| IBIS file 3599z.ibs created by s2ibis2 version 1.1
| North Carolina State University Electronics Research Laboratory  1995
[IBIS ver]   2.1
[File name]   v3599bc.ibs
[File Rev]   2.0
|1.0 : Original Version - Wei-Ling Chang
|2.0 : Replaced I/O and Input models with 70V659 ADC models - S.Kashyap 06/30/04
[Source]   Integrated Device Technology, Inc.
[Notes]   1.Temperatures: typ=25C, min=100C, max=0C 2.RRmp rates based
   on 50 ohm load. 3. Both inpad and iopad have 2 models each.
   (JTAG pins have one model.)
   iopad: standard 3.3V I/O model
   inpad: standard 3.3V input pad model
   iopad25: For 2.5V I/O supply
   inpad25: For 2.5V I/O supply.
   To use 2.%V models at any port, use iopad25 and inpad25
   as the model definition in pin defie section of the IBIS
   file.  JTAG pins only have models for 3.3V I/O voltage.
[Disclaimer] Integrated Device Technology, Inc. ("IDT") hereby grants the
   user of this IBIS model a non-exclusive, nontransferable
   license to use this IBIS model under the following terms. The
   user is granted this license only to use the IBIS model and is
   not granted rights to sell, copy (except as needed to run the
   IBIS model), rent, lease or sub-license the IBIS model in
   whole or in part, or in modified form to anyone. The User may
   modify the IBIS model to suit its specific applications, but
   rights to derivative works and such modifications shall belong
   to IDT. This IBIS model is provided on an AS IS" basis and IDT
   makes absolutely no warranty with respect to the information
   contained herein. IDT DISCLAIMS AND CUSTOMER WAIVES ALL
   WARRANTIES, EXPRESS AND IMPLIED, INCLUDING WARRANTIES OF
   MERCHANTABILITY AND FITNESS FOR A PARTICULAR PURPOSE. THE
   ENTIRE RISK AS TO QUALITY AND PERFORMANCE IS WITH THE USER
   ACCORDINGLY, IN NO EVENT SHALL IDT BE LIABLE FOR ANY DIRECT OR
   INDIRECT DAMAGES, WHETHER IN CONTRACT OR TORT, INCLUDING ANY
   LOST PROFITS OR OTHER INCIDENTAL, CONSEQUENTIAL, EXEMPLARY, OR
   PUNITIVE DAMAGES ARISING OUT OF THE USE OR APPLICATION OF THE
   IBIS model. Further, IDT reserves the right to make changes
   without notice to any product herein to improve reliability,
   function, or design. IDT does not convey any license under
   patent rights or any other intellectual property rights,
   including those of third parties. IDT is not obligated to
   provide maintenance or support for the licensed IBIS model.
[Copyright]   Copyright 2004, Integrated Device Technology, Inc. all rights
   reserved
|   Component idt70v3599z
[Component]   idt70v3599z
[Manufacturer]   Integrated Device Technology
[Package]
| BGA (BC256)
| variable   typ   min   max
R_pkg   54.00m   48.00m   60.00m
L_pkg   2.48nH   2.20nH   2.75nH
C_pkg   0.46pF   0.41pF   0.51pF
[Pin]  signal_name   model_name   R_pin   L_pin   C_pin
C2   io19l   iopad
D2   io19r   iopad
D3   io20l   iopad
D1   io20r   iopad
D5   vddql   POWER
E7   vss   GND
E2   io21l   iopad
E1   io21r   iopad
E3   io22l   iopad
F2   io22r   iopad
D7   vddqr   POWER
E8   vss   GND
F1   io23l   iopad
F3   io23r   iopad
G2   io24l   iopad
G1   io24r   iopad
D6   vddql   POWER
F6   vss   GND
G3   io25l   iopad
H2   io25r   iopad
H1   io26l   iopad
H3   io26r   iopad
G4   vddqr   POWER
G5   vss   GND
D4   vdd   POWER
E5   vdd   POWER
G6   vss   GND
E4   vddql   POWER
C3   vss   GND
J3   io27r   iopad
J1   io27l   iopad
J2   io28r   iopad
K3   io28l   iopad
H4   vddqr   POWER
H5   vss   GND
K1   io29r   iopad
K2   io29l   iopad
L3   io30r   iopad
L1   io30l   iopad
J4   vddql   POWER
J5   vss   GND
L2   io31r   iopad
M3   io31l   iopad
M1   io32r   iopad
M2   io32l   iopad
L4   vddqr   POWER
L6   vss   GND
N3   io33r   iopad
N1   io33l   iopad
N2   io34r   iopad
P2   io34l   iopad
P1   io35r   iopad
R1   io35l   iopad
N4   vdd   POWER
M7   vss   GND
P4   a16r   inpad
R5   a15r   inpad
T5   a14r   inpad
P5   a13r   inpad
R6   a12r   inpad
T6   a11r   inpad
P6   a10r   inpad
R7   a9r   inpad
T7   a8r   inpad
P7   a7r   inpad
R8   be3r#   inpad
T8   be2r#   inpad
P8   be1r#   inpad
P9   be0r#   inpad
T9   ce1r   inpad
R9   ce0r#   inpad
N13   vdd   POWER
M12   vdd   POWER
M9   vss   GND
M10   vss   GND
P10   clkr   inpad
T10   oer#   inpad
R10   rwr#   inpad
P11   adsr#   inpad
T11   cntenr#   inpad
R11   repeatr#  inpad
P12   a6r   inpad
T12   a5r   inpad
R12   a4r   inpad
P13   a3r   inpad
T13   a2r   inpad
R13   a1r   inpad
T14   a0r   inpad
M11   vdd   POWER
M8   vss   GND
M6   vdd   POWER
P14   io0l   iopad
P15   io0r   iopad
N12   vddql   POWER
L11   vss   GND
P16   io1l   iopad
N15   io1r   iopad
N14   io2l   iopad
N16   io2r   iopad
N10   vddqr   POWER
L10   vss   GND
M15   io3l   iopad
M14   io3r   iopad
M16   io4l   iopad
L15   io4r   iopad
N11   vddql   POWER
L9   vss   GND
L14   io5l   iopad
L16   io5r   iopad
K15   io6l   iopad
K14   io6r   iopad
K13   vddqr   POWER
K12   vss   GND
K16   io7l   iopad
J15   io7r   iopad
J16   io8l   iopad
J14   io8r   iopad
M13   vddql   POWER
K9   vss   GND
K10   vss   GND
K11   vss   GND
L12   vdd   POWER
M5   vdd   POWER
N9   vddqr   POWER
L8   vss   GND
H14   io9r   iopad
H15   io9l   iopad
H16   io10r   iopad
G14   io10l   iopad
L13   vddql   POWER
L7   vss   GND
G16   io11r   iopad
G15   io11l   iopad
F14   io12r   iopad
F16   io12l   iopad
J13   vddqr   POWER
J12   vss   GND
F15   io13r   iopad
E14   io13l   iopad
E16   io14r   iopad
E15   io14l   iopad
H13   vddql   POWER
H12   vss   GND
D14   io15r   iopad
D15   io15l   iopad
D16   io16r   iopad
C16   io16l   iopad
G12   vss   GND
F13   vddqr   POWER
C15   io17r   iopad
B15   io17l   iopad
L5   vdd   POWER
F11   vss   GND
F5   vdd   POWER
D13   vdd   POWER
A14   a0l   inpad
B13   a1l   inpad
A13   a2l   inpad
C13   a3l   inpad
B12   a4l   inpad
A12   a5l   inpad
C12   a6l   inpad
B11   repeatl#  inpad
A11   cntenl#   inpad
C11   adsl#   inpad
B10   rwl#   inpad
A10   oel#   inpad
C10   clkl   inpad
E9   vss   GND
E10   vss   GND
B14   vdd   POWER
E6   vdd   POWER
B9   ce0l   inpad
A9   ce1l   inpad
C9   be0l#   inpad
C8   be1l#   inpad
A8   be2l#   inpad
B8   be3l#   inpad
C7   a7l   inpad
A7   a8l   inpad
B7   a9l   inpad
C6   a10l   inpad
A6   a11l   inpad
B6   a12l   inpad
C5   a13l   inpad
A5   a14l   inpad
B5   a15l   inpad
C4   a16l   inpad
F9   vss   GND
E11   vdd   POWER
F10   vss   GND
B1   io18l   iopad
C1   io18r   iopad
D12   vddqr   POWER
F8   vss   GND
R14   optr   inpad
C14   optl   inpad
D11   vddqr   POWER
E13   vddqr   POWER
N5   vddqr   POWER
N6   vddqr   POWER
D8   vddqr   POWER
M4   vddqr   POWER
G13   vddql   POWER
F4   vddql   POWER
D9   vddql   POWER
D10   vddql   POWER
K4   vddql   POWER
N7   vddql   POWER
N8   vddql   POWER
E12   vdd   POWER
F12   vdd   POWER
F7   vss   GND
G7   vss   GND
G8   vss   GND
G9   vss   GND
G10   vss   GND
G11   vss   GND
H6   vss   GND
H7   vss   GND
H8   vss   GND
H9   vss   GND
H10   vss   GND
H11   vss   GND
J6   vss   GND
J7   vss   GND
J8   vss   GND
J9   vss   GND
J10   vss   GND
J11   vss   GND
K5   vss   GND
K6   vss   GND
K7   vss   GND
K8   vss   GND
P3   tms   inpadbs
T2   tck   inpadbs
R3   trst#   inpadbs
A2   tdi   inpadbs
B3   tdo   iopad
| in   in   dummy_model
| oe   oe   dummy_model
[Pin Mapping]  pulldown_ref   pullup_ref   gnd_clamp_ref   power_clamp_ref
C2  EXTGND   EXTVDDQ   EXTGND   EXTVDD
D2  EXTGND   EXTVDDQ   EXTGND   EXTVDD
D3  EXTGND   EXTVDDQ   EXTGND   EXTVDD
D1  EXTGND   EXTVDDQ   EXTGND   EXTVDD
D5  NC   EXTVDDQ
E7  EXTGND   NC
E2  EXTGND   EXTVDDQ   EXTGND   EXTVDD
E1  EXTGND   EXTVDDQ   EXTGND   EXTVDD
E3  EXTGND   EXTVDDQ   EXTGND   EXTVDD
F2  EXTGND   EXTVDDQ   EXTGND   EXTVDD
D7  NC   EXTVDDQ
E8  EXTGND   NC
F1  EXTGND   EXTVDDQ   EXTGND   EXTVDD
F3  EXTGND   EXTVDDQ   EXTGND   EXTVDD
G2  EXTGND   EXTVDDQ   EXTGND   EXTVDD
G1  EXTGND   EXTVDDQ   EXTGND   EXTVDD
D6  NC   EXTVDDQ
F6  EXTGND   NC
G3  EXTGND   EXTVDDQ   EXTGND   EXTVDD
H2  EXTGND   EXTVDDQ   EXTGND   EXTVDD
H1  EXTGND   EXTVDDQ   EXTGND   EXTVDD
H3  EXTGND   EXTVDDQ   EXTGND   EXTVDD
G4  NC   EXTVDDQ
G5  EXTGND   NC
D4  NC   EXTVDD
E5  NC   EXTVDD
G6  EXTGND   NC
E4  NC   EXTVDDQ
C3  EXTGND   NC
J3  EXTGND   EXTVDDQ   EXTGND   EXTVDD
J1  EXTGND   EXTVDDQ   EXTGND   EXTVDD
J2  EXTGND   EXTVDDQ   EXTGND   EXTVDD
K3  EXTGND   EXTVDDQ   EXTGND   EXTVDD
H4  NC   EXTVDDQ
H5  EXTGND   NC
K1  EXTGND   EXTVDDQ   EXTGND   EXTVDD
K2  EXTGND   EXTVDDQ   EXTGND   EXTVDD
L3  EXTGND   EXTVDDQ   EXTGND   EXTVDD
L1  EXTGND   EXTVDDQ   EXTGND   EXTVDD
J4  NC   EXTVDDQ
J5  EXTGND   NC
L2  EXTGND   EXTVDDQ   EXTGND   EXTVDD
M3  EXTGND   EXTVDDQ   EXTGND   EXTVDD
M1  EXTGND   EXTVDDQ   EXTGND   EXTVDD
M2  EXTGND   EXTVDDQ   EXTGND   EXTVDD
L4  NC   EXTVDDQ
L6  EXTGND   NC
N3  EXTGND   EXTVDDQ   EXTGND   EXTVDD
N1  EXTGND   EXTVDDQ   EXTGND   EXTVDD
N2  EXTGND   EXTVDDQ   EXTGND   EXTVDD
P2  EXTGND   EXTVDDQ   EXTGND   EXTVDD
P1  EXTGND   EXTVDDQ   EXTGND   EXTVDD
R1  EXTGND   EXTVDDQ   EXTGND   EXTVDD
N4  NC   EXTVDD
M7  EXTGND   NC
P4  EXTGND   EXTVDDQ   EXTGND   EXTVDD
R5  EXTGND   EXTVDDQ   EXTGND   EXTVDD
T5  EXTGND   EXTVDDQ   EXTGND   EXTVDD
P5  EXTGND   EXTVDDQ   EXTGND   EXTVDD
R6  EXTGND   EXTVDDQ   EXTGND   EXTVDD
T6  EXTGND   EXTVDDQ   EXTGND   EXTVDD
P6  EXTGND   EXTVDDQ   EXTGND   EXTVDD
R7  EXTGND   EXTVDDQ   EXTGND   EXTVDD
T7  EXTGND   EXTVDDQ   EXTGND   EXTVDD
P7  EXTGND   EXTVDDQ   EXTGND   EXTVDD
R8  EXTGND   EXTVDDQ   EXTGND   EXTVDD
T8  EXTGND   EXTVDDQ   EXTGND   EXTVDD
P8  EXTGND   EXTVDDQ   EXTGND   EXTVDD
P9  EXTGND   EXTVDDQ   EXTGND   EXTVDD
T9  EXTGND   EXTVDDQ   EXTGND   EXTVDD
R9  EXTGND   EXTVDDQ   EXTGND   EXTVDD
N13   NC   EXTVDD
M12   NC   EXTVDD
M9  EXTGND   NC
M10   EXTGND   NC
P10   EXTGND   EXTVDDQ   EXTGND   EXTVDD
T10   EXTGND   EXTVDDQ   EXTGND   EXTVDD
R10   EXTGND   EXTVDDQ   EXTGND   EXTVDD
P11   EXTGND   EXTVDDQ   EXTGND   EXTVDD
T11   EXTGND   EXTVDDQ   EXTGND   EXTVDD
R11   EXTGND   EXTVDDQ   EXTGND   EXTVDD
P12   EXTGND   EXTVDDQ   EXTGND   EXTVDD
T12   EXTGND   EXTVDDQ   EXTGND   EXTVDD
R12   EXTGND   EXTVDDQ   EXTGND   EXTVDD
P13   EXTGND   EXTVDDQ   EXTGND   EXTVDD
T13   EXTGND   EXTVDDQ   EXTGND   EXTVDD
R13   EXTGND   EXTVDDQ   EXTGND   EXTVDD
T14   EXTGND   EXTVDDQ   EXTGND   EXTVDD
M11   NC   EXTVDD
M8  EXTGND   NC
M6  NC   EXTVDD
P14   EXTGND   EXTVDDQ   EXTGND   EXTVDD
P15   EXTGND   EXTVDDQ   EXTGND   EXTVDD
N12   NC   EXTVDDQ
L11   EXTGND   NC
P16   EXTGND   EXTVDDQ   EXTGND   EXTVDD
N15   EXTGND   EXTVDDQ   EXTGND   EXTVDD
N14   EXTGND   EXTVDDQ   EXTGND   EXTVDD
N16   EXTGND   EXTVDDQ   EXTGND   EXTVDD
N10   NC   EXTVDDQ
L10   EXTGND   NC
M15   EXTGND   EXTVDDQ   EXTGND   EXTVDD
M14   EXTGND   EXTVDDQ   EXTGND   EXTVDD
M16   EXTGND   EXTVDDQ   EXTGND   EXTVDD
L15   EXTGND   EXTVDDQ   EXTGND   EXTVDD
N11   NC   EXTVDDQ
L9  EXTGND   NC
L14   EXTGND   EXTVDDQ   EXTGND   EXTVDD
L16   EXTGND   EXTVDDQ   EXTGND   EXTVDD
K15   EXTGND   EXTVDDQ   EXTGND   EXTVDD
K14   EXTGND   EXTVDDQ   EXTGND   EXTVDD
K13   NC   EXTVDDQ
K12   EXTGND   NC
K16   EXTGND   EXTVDDQ   EXTGND   EXTVDD
J15   EXTGND   EXTVDDQ   EXTGND   EXTVDD
J16   EXTGND   EXTVDDQ   EXTGND   EXTVDD
J14   EXTGND   EXTVDDQ   EXTGND   EXTVDD
M13   NC   EXTVDDQ
K9  EXTGND   NC
K10   EXTGND   NC
K11   EXTGND   NC
L12   NC   EXTVDD
M5  NC   EXTVDD
N9  NC   EXTVDDQ
L8  EXTGND   NC
H14   EXTGND   EXTVDDQ   EXTGND   EXTVDD
H15   EXTGND   EXTVDDQ   EXTGND   EXTVDD
H16   EXTGND   EXTVDDQ   EXTGND   EXTVDD
G14   EXTGND   EXTVDDQ   EXTGND   EXTVDD
L13   NC   EXTVDDQ
L7  EXTGND   NC
G16   EXTGND   EXTVDDQ   EXTGND   EXTVDD
G15   EXTGND   EXTVDDQ   EXTGND   EXTVDD
F14   EXTGND   EXTVDDQ   EXTGND   EXTVDD
F16   EXTGND   EXTVDDQ   EXTGND   EXTVDD
J13   NC   EXTVDDQ
J12   EXTGND   NC
F15   EXTGND   EXTVDDQ   EXTGND   EXTVDD
E14   EXTGND   EXTVDDQ   EXTGND   EXTVDD
E16   EXTGND   EXTVDDQ   EXTGND   EXTVDD
E15   EXTGND   EXTVDDQ   EXTGND   EXTVDD
H13   NC   EXTVDDQ
H12   EXTGND   NC
D14   EXTGND   EXTVDDQ   EXTGND   EXTVDD
D15   EXTGND   EXTVDDQ   EXTGND   EXTVDD
D16   EXTGND   EXTVDDQ   EXTGND   EXTVDD
C16   EXTGND   EXTVDDQ   EXTGND   EXTVDD
G12   EXTGND   NC
F13   NC   EXTVDDQ
C15   EXTGND   EXTVDDQ   EXTGND   EXTVDD
B15   EXTGND   EXTVDDQ   EXTGND   EXTVDD
L5  NC   EXTVDD
F11   EXTGND   NC
F5  NC   EXTVDD
D13   NC   EXTVDD
A14   EXTGND   EXTVDDQ   EXTGND   EXTVDD
B13   EXTGND   EXTVDDQ   EXTGND   EXTVDD
A13   EXTGND   EXTVDDQ   EXTGND   EXTVDD
C13   EXTGND   EXTVDDQ   EXTGND   EXTVDD
B12   EXTGND   EXTVDDQ   EXTGND   EXTVDD
A12   EXTGND   EXTVDDQ   EXTGND   EXTVDD
C12   EXTGND   EXTVDDQ   EXTGND   EXTVDD
B11   EXTGND   EXTVDDQ   EXTGND   EXTVDD
A11   EXTGND   EXTVDDQ   EXTGND   EXTVDD
C11   EXTGND   EXTVDDQ   EXTGND   EXTVDD
B10   EXTGND   EXTVDDQ   EXTGND   EXTVDD
A10   EXTGND   EXTVDDQ   EXTGND   EXTVDD
C10   EXTGND   EXTVDDQ   EXTGND   EXTVDD
E9  EXTGND   NC
E10   EXTGND   NC
B14   NC   EXTVDD
E6  NC   EXTVDD
B9  EXTGND   EXTVDDQ   EXTGND   EXTVDD
A9  EXTGND   EXTVDDQ   EXTGND   EXTVDD
C9  EXTGND   EXTVDDQ   EXTGND   EXTVDD
C8  EXTGND   EXTVDDQ   EXTGND   EXTVDD
A8  EXTGND   EXTVDDQ   EXTGND   EXTVDD
B8  EXTGND   EXTVDDQ   EXTGND   EXTVDD
C7  EXTGND   EXTVDDQ   EXTGND   EXTVDD
A7  EXTGND   EXTVDDQ   EXTGND   EXTVDD
B7  EXTGND   EXTVDDQ   EXTGND   EXTVDD
C6  EXTGND   EXTVDDQ   EXTGND   EXTVDD
A6  EXTGND   EXTVDDQ   EXTGND   EXTVDD
B6  EXTGND   EXTVDDQ   EXTGND   EXTVDD
C5  EXTGND   EXTVDDQ   EXTGND   EXTVDD
A5  EXTGND   EXTVDDQ   EXTGND   EXTVDD
B5  EXTGND   EXTVDDQ   EXTGND   EXTVDD
C4  EXTGND   EXTVDDQ   EXTGND   EXTVDD
F9  EXTGND   NC
E11   NC   EXTVDD
F10   EXTGND   NC
B1  EXTGND   EXTVDDQ   EXTGND   EXTVDD
C1  EXTGND   EXTVDDQ   EXTGND   EXTVDD
D12   NC   EXTVDDQ
F8  EXTGND   NC
R14   EXTGND   EXTVDDQ   EXTGND   EXTVDD
C14   EXTGND   EXTVDDQ   EXTGND   EXTVDD
D11   NC   EXTVDDQ
E13   NC   EXTVDDQ
N5  NC   EXTVDDQ
N6  NC   EXTVDDQ
D8  NC   EXTVDDQ
M4  NC   EXTVDDQ
G13   NC   EXTVDDQ
F4  NC   EXTVDDQ
D9  NC   EXTVDDQ
D10   NC   EXTVDDQ
K4  NC   EXTVDDQ
N7  NC   EXTVDDQ
N8  NC   EXTVDDQ
E12   NC   EXTVDD
F12   NC   EXTVDD
F7  EXTGND   NC
G7  EXTGND   NC
G8  EXTGND   NC
G9  EXTGND   NC
G10   EXTGND   NC
G11   EXTGND   NC
H6  EXTGND   NC
H7  EXTGND   NC
H8  EXTGND   NC
H9  EXTGND   NC
H10   EXTGND   NC
H11   EXTGND   NC
J6  EXTGND   NC
J7  EXTGND   NC
J8  EXTGND   NC
J9  EXTGND   NC
J10   EXTGND   NC
J11   EXTGND   NC
K5  EXTGND   NC
K6  EXTGND   NC
K7  EXTGND   NC
K8  EXTGND   NC
P3  EXTGND   EXTVDDQ   EXTGND   EXTVDD
T2  EXTGND   EXTVDDQ   EXTGND   EXTVDD
R3  EXTGND   EXTVDDQ   EXTGND   EXTVDD
A2  EXTGND   EXTVDDQ   EXTGND   EXTVDD
B3  EXTGND   EXTVDDQ   EXTGND   EXTVDD
| Models and submodels in the file (5): iopad (I/O), inpad (Input), inpadbs (Input), iopad25 (I/O), inpad25 (Input)
